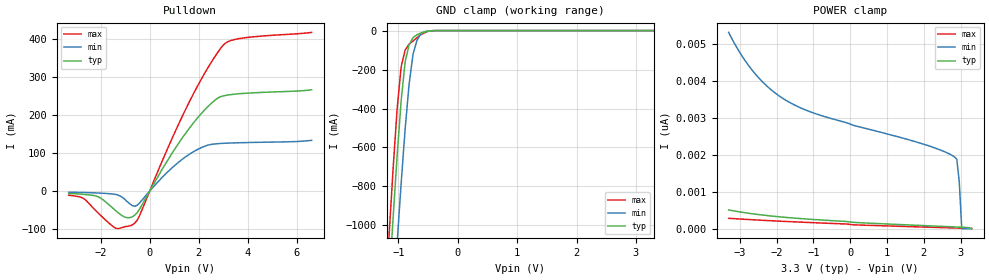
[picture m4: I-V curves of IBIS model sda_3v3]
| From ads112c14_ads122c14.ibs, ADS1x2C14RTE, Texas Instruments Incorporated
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|   Model sda_3v3
[Model] sda_3v3
Model_type I/O_open_drain
Polarity   Non-Inverting
Enable   Active-High
Vinl =  0.990V
Vinh =  2.310V
C_comp   4.000pF   2.000pF   8.000pF
[Model Spec]
Vinh   2.310V   2.100V   2.520V
Vinl   0.990V   0.900V   1.080V
[Temperature Range]   27.000   0.125k   -40.000
[Voltage Range]   3.300V   3.000V   3.600V
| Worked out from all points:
|   slope of the pulldown table from 0 to 0.495 V, typ, clamps not added: 8.89 ohm
|   GND clamp passes 1 mA (typ) near -0.45 V on its own axis
[Pulldown]
|Voltage   I(typ)   I(min)   I(max)
-3.3V     -5.999mA   -2.845mA   -10.81mA
-2.7V     -8.384mA   -3.559mA   -18.83mA
-2.1V     -14.71mA   -4.92mA    -57.29mA
-1.4V     -50.31mA   -8.452mA   -96.77mA
-700mV    -67.18mA   -38.11mA   -88.59mA
-400mV    -46.04mA   -30.25mA   -62.6mA
700mV     77.58mA    48.36mA    107.4mA
1.6V      163.9mA    96.24mA    232.5mA
2.4V      224mA      121.5mA    327.3mA
3V        250.4mA    125.7mA    384.1mA
3.9V      257.3mA    127.7mA    403.5mA
6.6V      266.5mA    133.6mA    417.4mA
[GND_clamp]
|Voltage   I(typ)   I(min)   I(max)
-3.3V     -8.723A    -8.387A    -9.129A
-1.156V   -1.293A    -1.738A    -1.045A
-1.089V   -960.1mA   -1.411A    -708.5mA
-1.022V   -644.8mA   -1.093A    -404.7mA
-955mV    -364.9mA   -789.3mA   -188.6mA
-888mV    -163.1mA   -511mA     -100.6mA
-821mV    -73.83mA   -277.9mA   -70.24mA
-754mV    -36.19mA   -121.9mA   -53.48mA
-687mV    -21.39mA   -49.48mA   -36.14mA
-620mV    -12.11mA   -16.45mA   -20.6mA
-419mV    -359.2uA   -386.2uA   -458.5uA
3.3V      0A         0A         0A
[POWER_clamp]
|Voltage   I(typ)   I(min)   I(max)
-3.3V     507.3pA    5.32nA     281.2pA
-2.931V   443.4pA    4.67nA     257.6pA
-2.529V   387pA      4.138nA    234.7pA
-2.127V   341.3pA    3.749nA    213.8pA
-1.658V   297.9pA    3.43nA     191.4pA
-854mV    239.4pA    3.089nA    156.3pA
1.96V     84.46pA    2.301nA    44.84pA
2.831V    46.86pA    1.948nA    19.41pA
2.898V    43.87pA    1.882nA    17.49pA
2.965V    40.84pA    1.266nA    15.58pA
3.032V    37.74pA    0A         13.67pA
3.3V      0A         0A         6.068pA
[Ramp]
| variable   typ   min   max
dV/dt_r   1.963/3.769n   1.776/3.649n   2.146/3.850n
dV/dt_f   1.963/0.189n   1.776/0.316n   2.146/0.131n
R_load = 1.000k
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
